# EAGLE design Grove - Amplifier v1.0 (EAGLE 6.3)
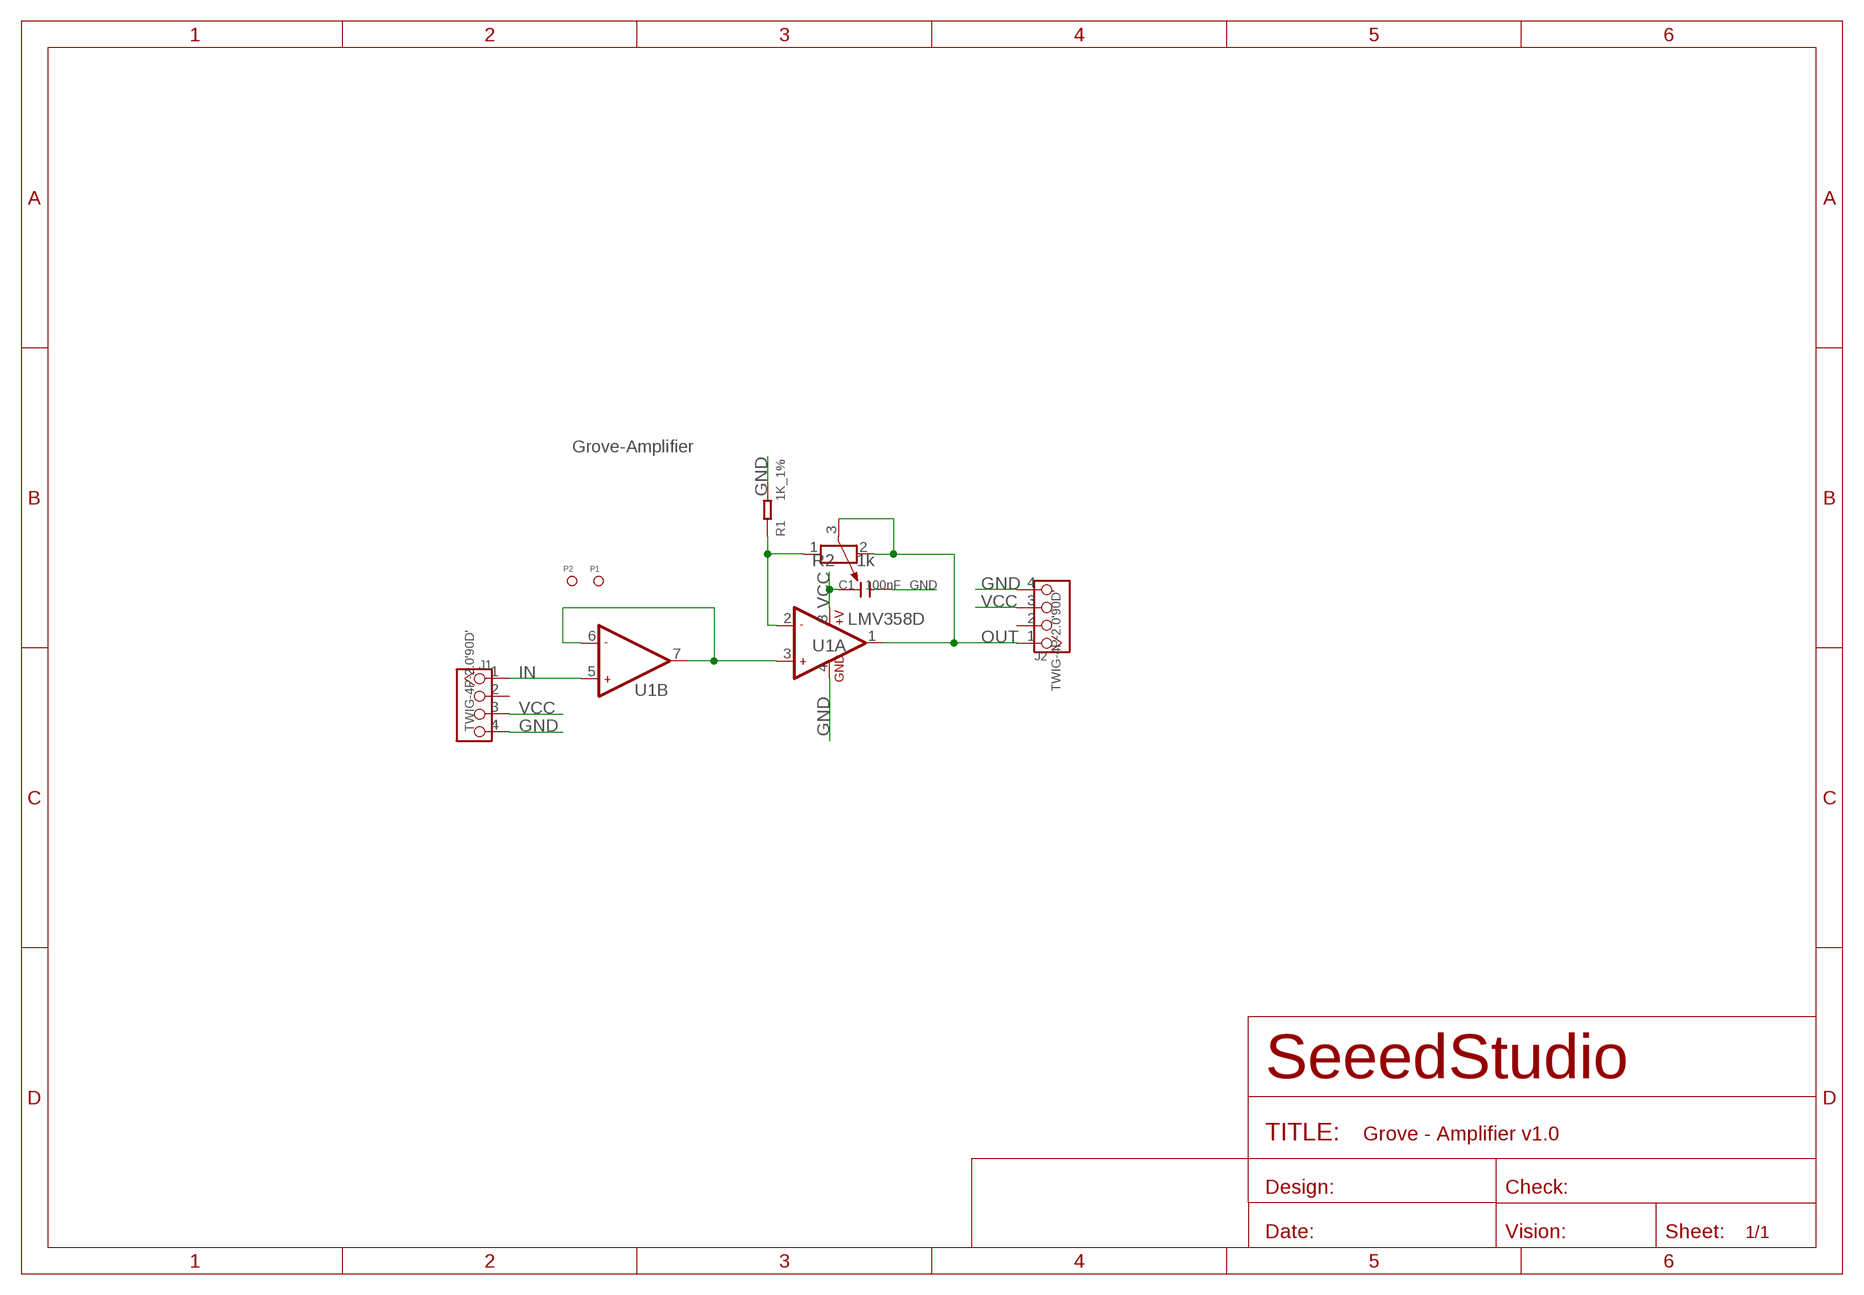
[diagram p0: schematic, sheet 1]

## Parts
C1  100nF  C-0603  [C0603]
J1  TWIG-4P-2.0'90D'  [4P-2.0-90D]
J2  TWIG-4P-2.0'90D'  [4P-2.0-90D]
P1  PAD-MARK  [ROUND-MARK-1.0]
P2  PAD-MARK  [ROUND-MARK-1.0]
R1  1K_1%  R-0603  [R0603]
R2  1k  R-POTENTIOMETER'3362'  [3P-SQUA-7X6.8]
U1  LMV358D  [SO08]

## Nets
GND: C1.2 J1.4 J2.4 R1.2 U1.4(A:GND)
IN: J1.1 U1.5(B:+IN2)
N$12: U1.3(A:+IN1) U1.6(B:-IN2) U1.7(B:OUT2)
N$16: R1.1 R2.1 U1.2(A:-IN1)
OUT: J2.1 R2.2 R2.3 U1.1(A:OUT1)
VCC: C1.1 J1.3 J2.3 U1.8(A:+V)
Unconnected: J1.2 J2.2

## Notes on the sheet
- Grove-Amplifier

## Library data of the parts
C1 = Discrete:C*: Ceramic Capacitors
J1 J2 = Connector:TWIG-4P-2.0
P1 P2 = Discrete:PAD-MARK; PARTNO: DNP
R1 = Discrete:R*
R2 = Discrete:R-POTENTIOMETER*: Potentiometer
U1 = IC:LMV358: General purpose LOW Voltage, Rail-to-Rail Output Amplifiers http://www.fairchildsemi.com/ds/LM/LMV358.pdf

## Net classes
0 default: width 0.152 mm, drill 0.305 mm, clearance 0.152 mm

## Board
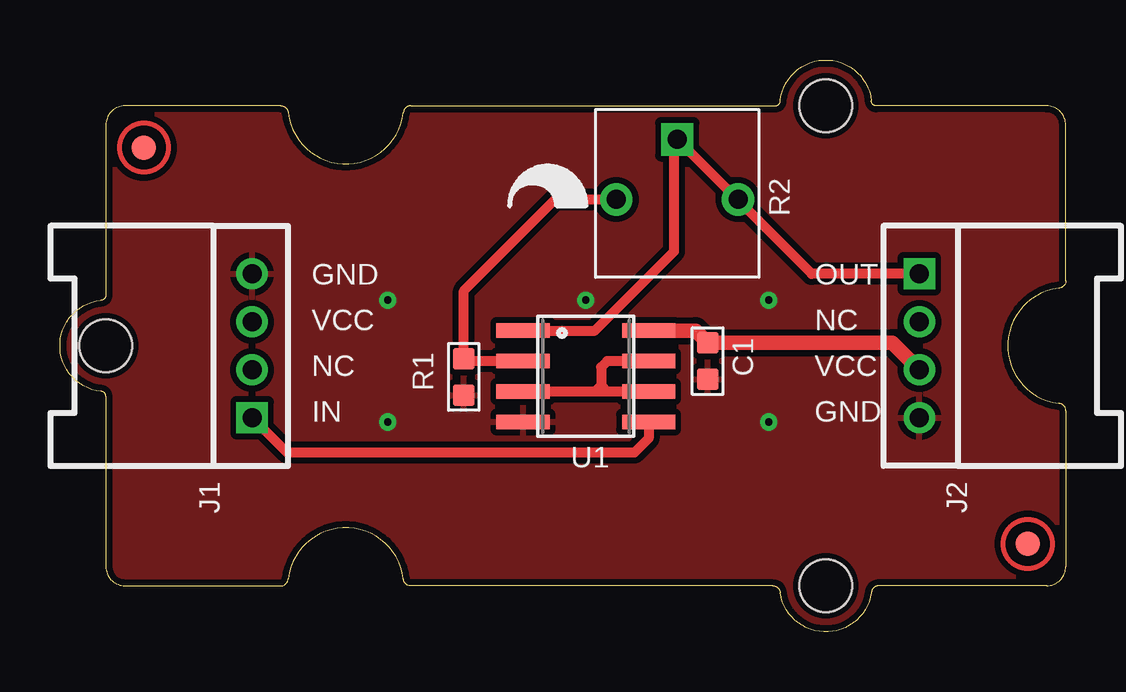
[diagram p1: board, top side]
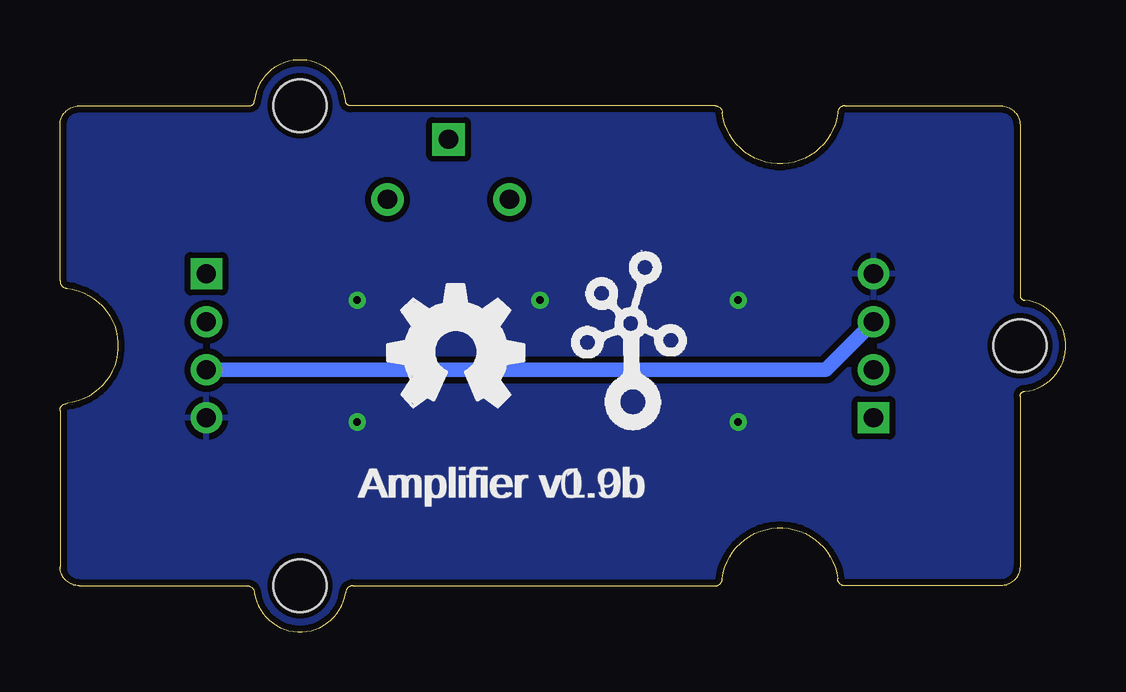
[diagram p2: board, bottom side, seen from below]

Size 41.91 x 23.83 mm. Coordinates in mm from the lower left corner, seen from the top.
Copper layers (1*16): Top 0.035mm / dielectric 1.5mm / Bottom 0.035mm
Design rules "default": minimum track width 10mil, minimum drill 12mil, track to track 8mil, track to pad 8mil, pad to pad 8mil, via to via 8mil, smd to smd 8mil, copper to edge 1mil, drill to drill 8mil, minimum pad ring 10mil, minimum via ring 8mil, stop-mask expansion 4mil, vias tented up to drill 25mil, thermal gap 10mil

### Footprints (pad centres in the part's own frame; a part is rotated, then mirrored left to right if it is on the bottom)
C0603 = smd 0.889 x 0.889: 1 -0.762,0; 2 0.762,0
4P-2.0-90D = drill 0.8 pad 1.27 square: 1 -3,0 | drill 0.8 pad 1.27: 2 -1,0; 3 1,0; 4 3,0
ROUND-MARK-1.0 = smd 1.016 x 1.016: P$1 0,0
R0603 = smd 0.889 x 0.889: 1 -0.762,0; 2 0.762,0
3P-SQUA-7X6.8 = drill 0.8 pad 1.35: 1 -2.54,-0.25; 2 2.54,-0.25 | drill 0.8 pad 1.35 square: 3 0,2.25
SO08 = smd 0.61 x 2.21: 1 -1.905,-2.616; 2 -0.635,-2.616; 3 0.635,-2.616; 4 1.905,-2.616; 5 1.905,2.616; 6 0.635,2.616; 7 -0.635,2.616; 8 -1.905,2.616
2U-DIM-W/DRILL = hole 2.2: -10,-10; -10,10; 20,0

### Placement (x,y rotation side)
C1  26.99,11.29 270 top
J1  8.01,11.92 90 top
J2  35.81,11.92 270 top
P1  3.49,20.18 0 top
P2  40.32,3.67 0 top
R1  16.82,10.62 270 top
R2  25.72,18.27 0 top
U1  21.91,10.65 270 top
U$1  [OSHW_FILLX200_NOTEXT]  28.26,9.39 0 bottom
U$3  [2U-DIM-W/DRILL]  21.91,11.92 180 top
U$4  [TWIGLOGO]  18.1,9.38 0 bottom

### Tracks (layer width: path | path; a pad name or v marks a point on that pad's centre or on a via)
GND  (via drill 0.3 pad 0.64)
  other vias: 29.53,13.83 29.53,8.75 13.65,8.75 13.65,13.83 21.91,13.83
  pour Bottom (isolate 0.254): -0.32,23.99 42.23,23.99 42.23,-0.78 -0.32,-0.78
  pour Top (isolate 0.254): -0.32,23.99 42.23,23.99 42.23,-0.78 -0.32,-0.78
IN
  Top 0.406: J1.1 9.45,7.48 23.94,7.48 24.52,8.06 U1.5
N$12
  Top 0.406: U1.6 22.8,10.02 | 22.8,10.02 22.54,10.02 | 22.54,10.02 22.29,10.02 | 22.29,10.02 U1.3 | U1.7 22.8,11.29 22.54,11.03 22.54,10.27 | 22.54,10.27 22.54,10.02 | 22.29,10.02 22.54,10.27 | 22.54,10.27 22.8,10.02
N$16
  Top 0.406: R1.1 16.92,11.29 U1.2 16.83,11.29 16.83,14.21 20.64,18.02 R2.1
OUT
  Top 0.406: J2.1 31.32,14.92 28.26,17.98 | 28.26,17.98 R2.3 25.59,20.39 25.59,15.86 22.29,12.56 U1.1 | R2.2 28.26,17.98
VCC
  Top 0.61: U1.8 26.48,12.56 C1.1 34.68,12.05 J2.3
  Bottom 0.61: J2.3 10.01,10.92 J1.3

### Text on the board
tPlace: GND | OUT | VCC | NC | NC | VCC | IN | GND
bPlace: Amplifier v1.0b
bNames: Amplifier v0.9b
